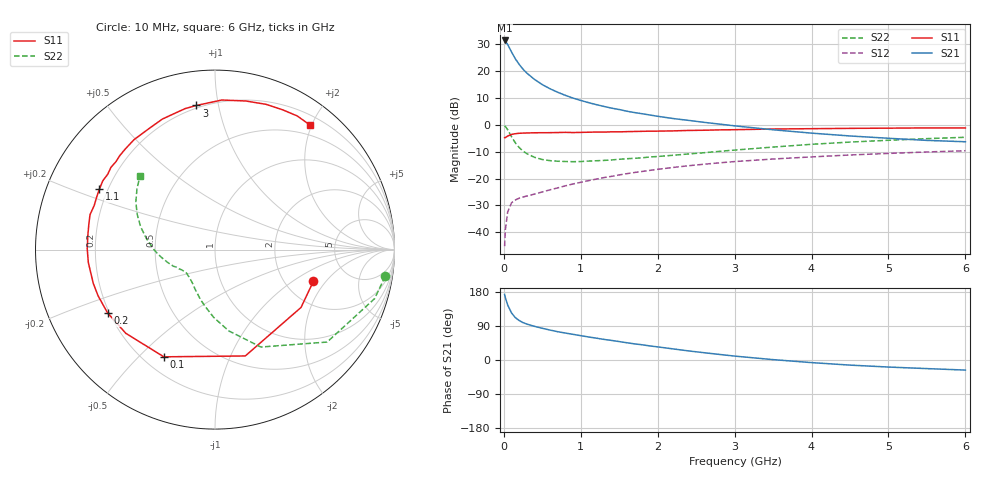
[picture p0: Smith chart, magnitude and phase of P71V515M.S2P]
! SIEMENS Small Signal Semiconductors
! BFP196
! Si NPN RF Bipolar Junction Transistor in SOT143
! VCE = 1.5 V  IC = 15 mA
! Common Emitter S-Parameters:  May  1996
# GHz  S  MA  R  50
!  f  S11  S21  S12  S22
! GHz  MAG  ANG  MAG  ANG  MAG  ANG  MAG  ANG
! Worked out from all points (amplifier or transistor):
!   36 points, 10 MHz to 6 GHz, reference 50 ohm
!   highest |S21| = 31.4 dB at 10 MHz (marker M1)
!   |S21| within 3 dB of that: start of sweep to 76.76 MHz
!   unconditionally stable (mu >= 1): 751.2 MHz to 3.411 GHz
!   at 250 MHz: K = 0.52, MSG = 23.8 dB, |S12| = -26.9 dB
!   at 1.4 GHz: K = 1.13, MAG = 10.5 dB, |S12| = -19.2 dB
!   at 6 GHz: K = 0.99, MSG = 1.7 dB, |S12| = -9.7 dB
!   S11 on the Smith chart (normalised r, x): 10 MHz: 2.84, -1.50; 100 MHz: 0.28, -0.60; 200 MHz: 0.19, -0.26; 1.1 GHz: 0.17, +0.24; 3 GHz: 0.18, +0.86; 6 GHz: 0.34, +1.97
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0.01  0.576 -17.8  37.12 172.9  0.0055 83.2  0.9601 -8.9
0.02  0.5776 -33.9  35.8 164.3  0.0112 76.4  0.9301 -17.1
0.05  0.6161 -74.1  31.2 145.1  0.0239 60.1  0.8097 -39.5
0.1  0.6619 -115.5  22.64 124.0  0.0353 45.1  0.5999 -64.8
0.15  0.6815 -136.8  16.85 111.7  0.0398 38.4  0.4593 -80.4
0.2  0.6948 -149.5  13.28 104.1  0.0431 36.5  0.377 -91.2
0.25  0.7005 -158.5  10.81 98.6  0.0453 36.4  0.3226 -99.6
0.3  0.7038 -164.5  9.134 94.7  0.0472 37.2  0.2898 -106.2
0.4  0.7095 -174.2  6.962 88.7  0.0513 39.1  0.2475 -116.5
0.5  0.7119 179.6  5.586 83.7  0.0562 41.1  0.2254 -123.8
0.6  0.7129 173.6  4.685 79.0  0.0616 43.4  0.215 -129.5
0.7  0.7172 168.4  4.03 74.7  0.0669 44.9  0.2096 -133.9
0.9  0.7165 160.0  3.137 67.7  0.0792 47.3  0.2056 -140.4
1.1  0.727 152.3  2.586 60.8  0.0912 48.3  0.2108 -144.6
1.3  0.7303 144.9  2.196 54.4  0.104 48.1  0.2171 -148.7
1.6  0.7453 135.4  1.788 45.5  0.1231 47.2  0.2335 -154.0
2.2  0.7695 117.8  1.307 29.3  0.1605 42.3  0.2707 -164.1
3  0.8096 97.4  0.955 10.3  0.2066 33.3  0.338 -179.5
3.5  0.8343 87.4  0.807 1.0  0.2306 27.3  0.3847 171.3
4.5  0.8578 70.7  0.619 -13.5  0.274 16.1  0.4761 155.6
5.5  0.8743 58.4  0.512 -22.7  0.3118 5.1  0.5522 141.9
6  0.8728 52.7  0.483 -26.6  0.3289 -0.8  0.5852 135.5
